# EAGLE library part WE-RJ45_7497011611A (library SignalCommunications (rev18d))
WE-RJ45 LAN Transformer Order Code 749701611A Design THT xBase-T 10/100 Base-T Ports 1x1 Application Standard Tab Position UP LED (Left-Right) Yellow-Green-ORANGE EMI Fingers No Details see: http://katalog.we-online.de/en/pbs/WE-LAN-RJ45 Created by Yingchun Shan 2016 (C) Wurth Elektronik
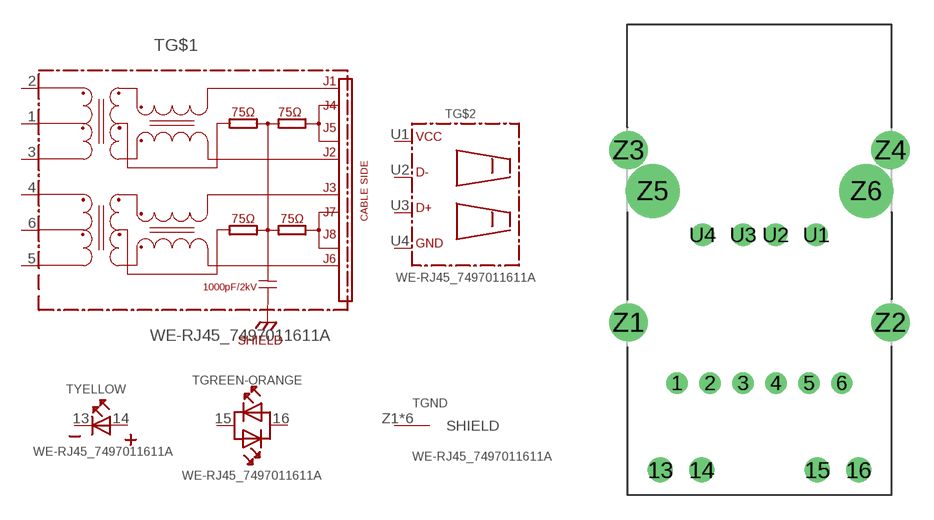
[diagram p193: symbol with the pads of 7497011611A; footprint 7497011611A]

Designator prefix T; gates G$1=7497011611A YELLOW=LED_2PIN GREEN-ORANGE=LED_DOUB G$2=USB2.0-1 GND=SHIELD

## WE-RJ45_7497011611A  [7497011611A]
1  G$1:1
2  G$1:2
3  G$1:3
4  G$1:4
5  G$1:5
6  G$1:6
13  YELLOW:K  pas
14  YELLOW:A  pas
15  GREEN-ORANGE:AK1  pas
16  GREEN-ORANGE:AK2  pas
U1  G$2:VUSB  pwr
U2  G$2:D-
U3  G$2:D+
U4  G$2:GND  pwr
Z1  GND:SHIELD  pas
Z2  GND:SHIELD  pas
Z3  GND:SHIELD  pas
Z4  GND:SHIELD  pas
Z5  GND:SHIELD  pas
Z6  GND:SHIELD  pas

## Footprint 7497011611A (pad centres in mm)
drill 0.8: 1 -5.07,-3.73; 2 -3.042,-3.73; 3 -1.014,-3.73; 4 1.014,-3.73; 5 3.042,-3.73; 6 5.07,-3.73
drill 1.02: 13 -6.1,-9.08; 14 -3.56,-9.08; 15 3.56,-9.08; 16 6.1,-9.08
drill 0.9: U1 3.5,5.41; U2 1,5.41; U3 -1,5.41; U4 -3.5,5.41
drill 1.57: Z1 -8.06,0; Z2 8.06,0; Z3 -8.06,10.62; Z4 8.06,10.62
drill 2.31: Z5 -6.57,8.11; Z6 6.57,8.11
